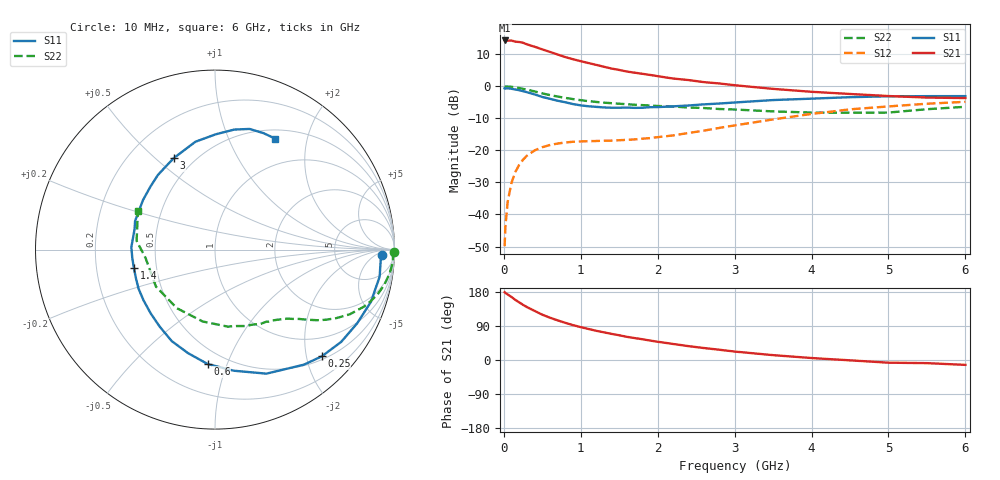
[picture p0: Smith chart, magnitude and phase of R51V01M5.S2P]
! SIEMENS Small Signal Semiconductors
! BFR183
! Si NPN RF Bipolar Junction Transistor in SOT23
! VCE = 1 V  IC = 1.5 mA
! Common Emitter S-Parameters:  May  1996
# GHz  S  MA  R  50
!  f  S11  S21  S12  S22
! GHz  MAG  ANG  MAG  ANG  MAG  ANG  MAG  ANG
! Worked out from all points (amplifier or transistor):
!   36 points, 10 MHz to 6 GHz, reference 50 ohm
!   highest |S21| = 14.3 dB at 10 MHz (marker M1)
!   |S21| within 3 dB of that: start of sweep to 527.2 MHz
!   unconditionally stable (mu >= 1): 1.459 GHz to 3.132 GHz
!   at 250 MHz: K = 0.20, MSG = 18.2 dB, |S12| = -22.9 dB
!   at 1.4 GHz: K = 0.98, MSG = 11.3 dB, |S12| = -16.9 dB
!   at 6 GHz: K = 0.97, MSG = 0.6 dB, |S12| = -4.8 dB
!   S11 on the Smith chart (normalised r, x): 10 MHz: 23, -11; 250 MHz: 0.56, -2.30; 600 MHz: 0.40, -0.86; 1.4 GHz: 0.37, -0.10; 3 GHz: 0.39, +0.58; 6 GHz: 0.61, +1.50
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0.01  0.9327 -2.0  5.203 178.9  0.0032 88.9  0.9966 -0.7
0.02  0.925 -3.8  5.101 177.1  0.0064 87.3  0.9915 -1.5
0.05  0.9297 -9.3  5.164 173.0  0.0159 86.1  0.9935 -3.9
0.1  0.9163 -18.5  5.18 166.2  0.0314 79.2  0.982 -7.8
0.15  0.8921 -27.5  4.98 158.6  0.0462 74.1  0.9643 -11.6
0.2  0.8709 -36.2  4.923 152.1  0.0596 69.8  0.9423 -15.0
0.25  0.8412 -45.0  4.785 145.5  0.0718 64.5  0.9142 -18.3
0.3  0.8102 -52.3  4.523 139.7  0.0827 60.7  0.888 -21.0
0.4  0.7481 -67.5  4.152 129.6  0.1 53.6  0.8334 -25.6
0.5  0.6825 -81.3  3.776 119.5  0.1123 47.9  0.7758 -29.5
0.6  0.6385 -93.7  3.447 111.6  0.1214 43.6  0.7296 -32.4
0.8  0.5639 -115.3  2.86 98.0  0.133 37.2  0.6598 -36.4
0.9  0.5285 -125.6  2.649 92.0  0.1364 35.5  0.6323 -38.0
1.1  0.4885 -144.5  2.31 81.9  0.1395 33.7  0.5878 -41.1
1.4  0.4632 -167.4  1.896 68.9  0.1421 34.0  0.5459 -45.2
1.9  0.4728 160.4  1.508 51.3  0.1556 40.2  0.5013 -53.1
2.2  0.487 145.4  1.324 42.3  0.1712 43.9  0.4849 -58.8
3  0.5595 114.1  1.041 22.3  0.2454 48.1  0.4349 -80.6
3.5  0.6108 100.3  0.913 12.8  0.3046 45.2  0.4063 -99.7
4.5  0.6773 80.9  0.76 -0.9  0.4374 32.6  0.3882 -148.0
5.5  0.7028 67.4  0.668 -8.3  0.5352 17.8  0.4395 173.6
6  0.7035 61.6  0.656 -12.9  0.573 8.6  0.4794 153.6
